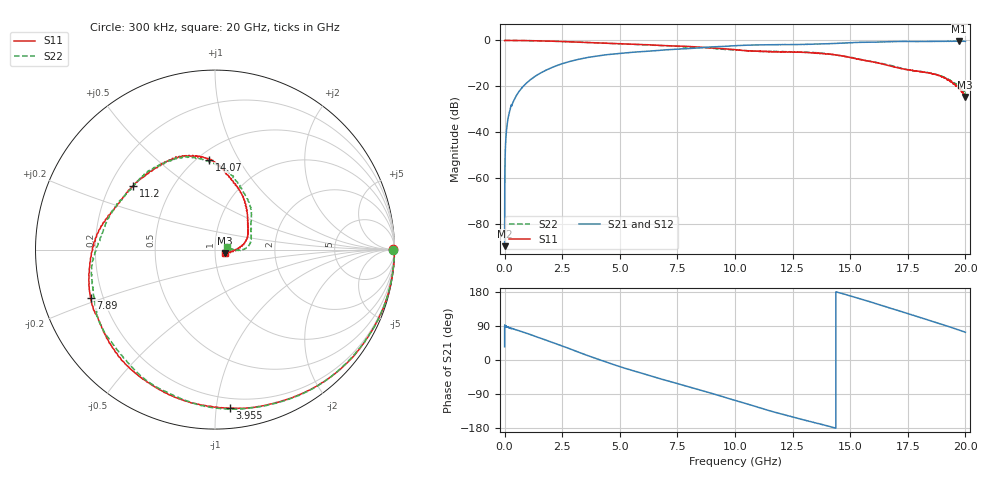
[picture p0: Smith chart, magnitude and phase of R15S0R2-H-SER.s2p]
!{R15S0R2}
!Johanson Technology Inc.
!www.johansontechnology.com
!Test Board Conditions:
!Substrate Type  RO4350B
!Substrate Thickness  20 mil
!Substrate Dk  3.66
!TL Type: GCPW
!TL Trace Width  34 mil
!TL Gap  10 mil
!Electrode orientation  Horizontal
!DUT TOPOLOGY	SERIES
!Mounting Pad LxW  26x52 mil
! Created Sat Feb  6 12:04:06 2021
# hz S ma R 50
! 2 Port Network Data from SP1.SP block
! freq  magS11  angS11  magS21  angS21  magS12  angS12  magS22  angS22
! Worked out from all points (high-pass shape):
!   20001 points, 300 kHz to 20 GHz, reference 50 ohm
!   highest |S21| = -0.32 dB at 19.73 GHz (marker M1); lowest = -89.7 dB at 300 kHz (marker M2)
!   |S21| within 3 dB of the highest: 8.282514 GHz to 8.288065 GHz (5.551 MHz wide, 0.067 % of centre); 8.293 GHz to end of sweep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
!   lowest |S11| = -24.6 dB at 19.99 GHz (marker M3), VSWR 1.12, Z = 55.7 - j2.36 ohm
!   |S11| at or under -10 dB: 16.29159 GHz to 16.29288 GHz (1.289 MHz wide, 0.00791 % of centre); 16.29 GHz to end of sweep
!   |S22| runs from -23.2 to 0.0 dB; largest |S21 - S12| = 0.018
!   S11 on the Smith chart (normalised r, x): 300 kHz: open; 3.955 GHz: 0.13, -1.09; 7.89 GHz: 0.15, -0.18; 11.2 GHz: 0.30, +0.32; 14.07 GHz: 0.57, +0.76; 20 GHz: 1.12, -0.05
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300000  0.9929 0.1  3.272e-05 35.2  2.93e-05 133.6  0.9925 -0.0
1.033e8  0.9989 -2.2  0.01378 87.7  0.01386 87.5  0.9999 -2.2
1.463e8  0.9998 -3.1  0.01943 86.8  0.01953 86.5  0.9995 -3.0
2.773e8  0.9988 -6.1  0.03699 83.3  0.03715 83.4  0.999 -6.1
5.383e8  0.9973 -10.9  0.06606 78.8  0.06629 79.0  0.9976 -10.8
1.5413e9  0.9795 -32.0  0.1924 57.9  0.193 57.9  0.979 -31.9
3.3343e9  0.9135 -71.3  0.3996 17.8  0.4011 17.9  0.9126 -72.6
3.9553e9  0.8873 -84.7  0.4552 4.2  0.4548 4.1  0.8891 -86.4
5.4463e9  0.8301 -115.6  0.5465 -25.8  0.5453 -25.8  0.8278 -115.4
6.6673e9  0.7852 -138.2  0.6056 -47.9  0.6073 -47.7  0.7747 -137.0
7.8903e9  0.7433 -158.9  0.6618 -69.1  0.6666 -69.0  0.7238 -158.6
1.00003e10  0.6311 164.1  0.7682 -106.6  0.7715 -106.5  0.6216 164.2
1.12023e10  0.5782 141.9  0.8008 -128.4  0.8084 -128.8  0.5748 141.6
1.33343e10  0.5383 103.4  0.8291 -163.6  0.8232 -163.6  0.5435 110.0
1.40703e10  0.5029 93.5  0.8513 -174.8  0.8433 -175.2  0.505 97.3
1.53633e10  0.389 74.7  0.9058 162.7  0.8969 163.0  0.3961 71.6
1.66673e10  0.2845 51.1  0.9408 138.2  0.9377 138.9  0.2936 46.4
1.77853e10  0.2182 32.4  0.9514 117.1  0.9489 117.1  0.217 22.6
1.88143e10  0.1732 14.6  0.9554 97.3  0.9557 97.6  0.1761 3.7
1.97253e10  0.08788 -10.2  0.9641 78.9  0.9607 79.3  0.09789 1.7
1.99913e10  0.05859 -21.1  0.9617 73.4  0.9591 73.4  0.07083 11.6
2e10  0.0592 -20.4  0.9584 73.2  0.959 73.3  0.06985 12.2
